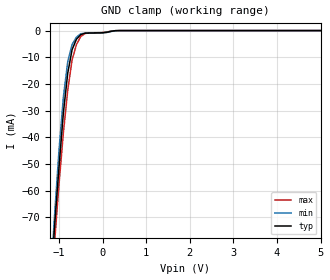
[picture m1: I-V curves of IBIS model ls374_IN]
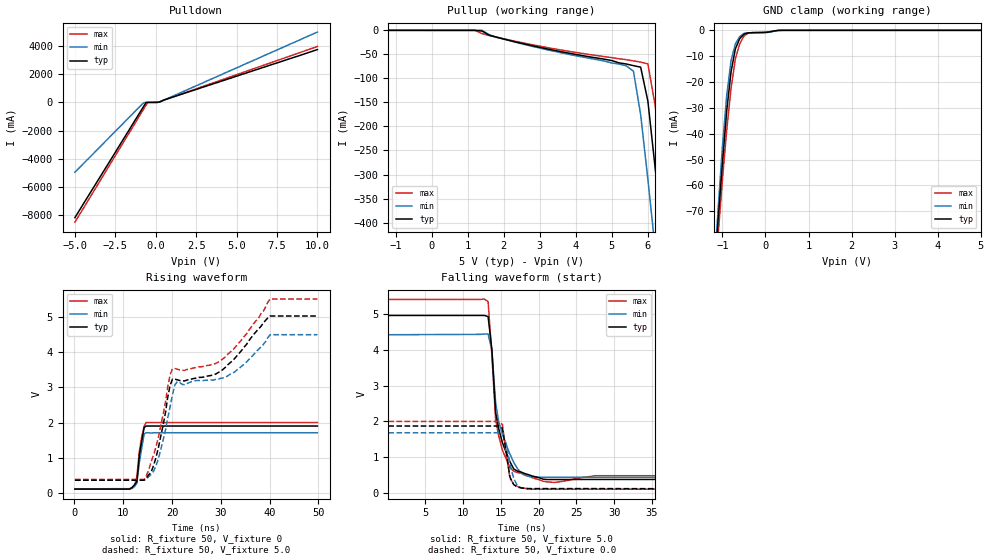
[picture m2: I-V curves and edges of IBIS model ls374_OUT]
| TEXAS INSTRUMENTS INCORPORATED
| Standard Linear and Logic Group
| IBIS Model of SN74LS374
| OCTAL D-TYPE TRANSPARENT LATCHES AND EDGE-TRIGGERED FLIP-FLOPS
| SOP 20-pin (NS), SSOP 20-pin (DB)
[IBIS Ver]   3.2
[Comment Char]  |_char
[File Name]   sn74ls374.ibs
[File Rev]   2.1 I_die
[Date]   November 18, 2004
[Source]   File originated at Texas Instruments, Inc.
[Notes]   The following is a sample IBIS file for the LS374.
   - FILE REV HISTORY
   - 2.1 Re-Release IBIS file on 11/19/04
   - Power clamp data deleted as there is no power-clamp diode
|   - All test data contained in this file are derived from
|   actual measurements.
|   - File created by Nobuhisa Ohtsubo, SLL Product Engineering.
[Disclaimer] Property of Texas Instruments Incorporated.  Unauthorized
   reproduction and/or distribution is strictly prohibited.
   This product is protected under copyright law.
   Created 2000, (C) Copyright 2000, Texas Instruments Inc.,
   All Rights Reserved.
   UNLESS THERE IS A SIGNED, WRITTEN AGREEMENT TO THE
   CONTRARY, TEXAS INSTRUMENTS () IS PROVIDING THE IBIS
   MODELS  AND WITHOUT ANY WARRANTY, EXPRESSED OR
   IMPLIED.  TI assumes no liability for:
   1) the accuracy of the IBIS models provided to your
   company;
   2) the proper functioning of these IBIS Models in your
   design or for any resulting applications; or
   3) infringement of patents, copyrights or intellectual
   property rights resulting from your use of these IBIS
   models.
   TI provides IBIS Models as a service to our customers.
   You and your company shall not distribute, sell or give
   these models to anyone else without prior written
   permission from TI.
   TI reserves the right to make changes to our products or
   to discontinue any semiconductor product or service
   without notice, and advises our customers to obtain the
   latest version of relevant information to verify, before
   placing orders, that the information being relied on is
   current.
   Please be aware that your receipt and use of the IBIS
   information provided shall serve as acceptance of these
   terms and conditions.  If you do not accept these terms,
   you should return or destroy the IBIS models and any
   other accompanying information immediately.
|   Component LS374_NS
[Component]   ls374_NS
[Manufacturer]  Texas Instruments, Inc.
[Package]
|   typ   min   max
R_pkg   0.044   0.029   0.058
L_pkg   3.666nH   2.317nH   5.115nH
C_pkg   0.548pF   0.316pF   0.725pF
[Pin]   signal_name   model_name   R_pin   L_pin   C_pin
1   OC_NOT   ls374_IN   0.058   5.115nH   0.725pF
2   1Q   ls374_OUT   0.053   4.591nH   0.724pF
3   1D   ls374_IN   0.049   3.754nH   0.572pF
4   2D   ls374_IN   0.029   2.549nH   0.388pF
5   2Q   ls374_OUT   0.031   2.317nH   0.316pF
6   3Q   ls374_OUT   0.031   2.317nH   0.316pF
7   3D   ls374_IN   0.029   2.556nH   0.399pF
8   4D   ls374_IN   0.049   3.754nH   0.579pF
9   4Q   ls374_OUT   0.053   4.591nH   0.724pF
10   GND   GND   0.058   5.115nH   0.725pF
11   CLK   ls374_IN   0.058   5.115nH   0.725pF
12   5Q   ls374_OUT   0.053   4.591nH   0.724pF
13   5D   ls374_IN   0.049   3.754nH   0.579pF
14   6D   ls374_IN   0.029   2.557nH   0.399pF
15   6Q   ls374_OUT   0.031   2.317nH   0.316pF
16   7Q   ls374_OUT   0.031   2.317nH   0.316pF
17   7D   ls374_IN   0.029   2.557nH   0.399pF
18   8D   ls374_IN   0.049   3.754nH   0.579pF
19   8Q   ls374_OUT   0.053   4.591nH   0.724pF
20   VCC   POWER   0.058   5.115nH   0.725pF
|   Component LS374_DB
[Component]   ls374_DB
[Manufacturer]  Texas Instruments, Inc.
[Package]
|   typ   min   max
R_pkg   0.040   0.035   0.051
L_pkg   3.495nH   3.035nH   4.314nH
C_pkg   0.420pF   0.346pF   0.502pF
[Pin]   signal_name   model_name   R_pin   L_pin   C_pin
1   OC_NOT   ls374_IN   0.049   4.310nH   0.502pF
2   1Q   ls374_OUT   0.048   3.903nH   0.487pF
3   1D   ls374_IN   0.035   3.189nH   0.396pF
4   2D   ls374_IN   0.035   3.036nH   0.347pF
5   2Q   ls374_OUT   0.035   3.035nH   0.367pF
6   3Q   ls374_OUT   0.035   3.035nH   0.367pF
7   3D   ls374_IN   0.035   3.036nH   0.347pF
8   4D   ls374_IN   0.035   3.189nH   0.397pF
9   4Q   ls374_OUT   0.047   3.899nH   0.488pF
10   GND   GND   0.051   4.314nH   0.500pF
11   CLK   ls374_IN   0.051   4.314nH   0.500pF
12   5Q   ls374_OUT   0.047   3.899nH   0.488pF
13   5D   ls374_IN   0.035   3.189nH   0.397pF
14   6D   ls374_IN   0.035   3.036nH   0.346pF
15   6Q   ls374_OUT   0.035   3.035nH   0.367pF
16   7Q   ls374_OUT   0.035   3.035nH   0.367pF
17   7D   ls374_IN   0.035   3.036nH   0.346pF
18   8D   ls374_IN   0.035   3.189nH   0.397pF
19   8Q   ls374_OUT   0.047   3.899nH   0.488pF
20   VCC   POWER   0.051   4.314nH   0.502pF
| Models and submodels in the file (2): ls374_IN (Input), ls374_OUT (3-state)
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|   Model LS374_IN
[Model]   ls374_IN
Model_type  Input
Polarity   Inverting
Vinl = 0.8
Vinh = 2.0
| variable   typ   min   max
C_comp   1.33pf   1.00pf   1.66pf
[Temperature Range]   25   0   70
[Voltage Range]   5.0   4.75   5.25
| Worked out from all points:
|   GND clamp passes 1 mA (typ) near -0.41 V on its own axis
[GND Clamp]
|   Voltage   I(typ)   I(min)   I(max)
-5V       -1.19A     -1.28A     -1.1A
-1.2V     -97.9mA    -94.9mA    -103mA
-1.1V     -73mA      -68.8mA    -79.1mA
-1V       -51.2mA    -44.9mA    -57.6mA
-900mV    -30.9mA    -25mA      -38.4mA
-800mV    -16mA      -11.7mA    -22.4mA
-700mV    -7.17mA    -5.25mA    -11mA
-600mV    -3.23mA    -2.46mA    -5.25mA
-500mV    -1.49mA    -1.17mA    -2.19mA
-400mV    -972uA     -958uA     -1.08mA
300mV     -31.8uA    -42.7uA    -27.7uA
5V        848pA      59.6pA     3.3nA
|   Model LS374_OUT
[Model]   ls374_OUT
Model_type  3-state
Polarity   Non-Inverting
Enable   Active-Low
Vmeas = 1.3v
Cref = 0pf
| variable   typ   min   max
C_comp   5.8pf   4.35pf   7.25pf
[Temperature Range]   25   0   70
[Voltage Range]   5.0   4.5   5.5
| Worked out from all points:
|   slope of the pulldown table from 0 to 0.75 V, typ, clamps not added: 2.87 ohm
|   GND clamp passes 1 mA (typ) near -0.41 V on its own axis
|   rising waveform, R_fixture 50, V_fixture 0: 20-80 % time 983ps typ, 1ns min, 1.02ns max; typ from 0.112 V to 1.9 V
|   falling waveform, R_fixture 50, V_fixture 5.0: 20-80 % time 1.62ns typ, 1.98ns min, 1.25ns max; typ from 4.97 V to 0.373 V
|   rising waveform, R_fixture 50, V_fixture 5.0: 20-80 % time 17.3ns typ, 17.3ns min, 18.1ns max; typ from 0.364 V to 5.02 V
|   falling waveform, R_fixture 50, V_fixture 0.0: 20-80 % time 763ps typ, 977ps min, 769ps max; typ from 1.87 V to 0.111 V
[Pulldown]
|   Voltage   I(typ)   I(min)   I(max)
-5V       -8.18A     -4.96A     -8.5A
-800mV    -386mA     -83.9mA    -577mA
-600mV    -14.5mA    -7.73mA    -200mA
-500mV    -6.86mA    -4.9mA     -11.3mA
100mV     -2.6mA     -3.4mA     -1.45mA
300mV     56.8mA     50mA       60.2mA
10V       3.74A      4.98A      3.96A
[Pullup]
|   Voltage   II(typ)   I(min)   I(max)
-5V       2.751uA    649.5nA    18.57uA
1.4V      -1.523mA   -61.48uA   -6.907mA
2.6V      -28.75mA   -29.78mA   -27.07mA
5.4V      -70.02mA   -73.84mA   -61.06mA
5.6V      -73.5mA    -85mA      -63.58mA
5.8V      -76.68mA   -175.9mA   -66.03mA
6V        -147.2mA   -309.9mA   -69.96mA
6.2V      -285.1mA   -453mA     -155.4mA
6.4V      -418.1mA   -591.7mA   -267.9mA
6.6V      -548.4mA   -727.9mA   -387.4mA
6.8V      -675.6mA   -862.2mA   -504.6mA
10V       -2.654A    -3.011A    -2.322A
[GND Clamp]
|   Voltage   I(typ)   I(min)   I(max)
-5V       -1.19A     -1.28A     -1.1A
-1.2V     -97.9mA    -94.9mA    -103mA
-1.1V     -73mA      -68.8mA    -79.1mA
-1V       -51.2mA    -44.9mA    -57.6mA
-900mV    -30.9mA    -25mA      -38.4mA
-800mV    -16mA      -11.7mA    -22.4mA
-700mV    -7.17mA    -5.25mA    -11mA
-600mV    -3.23mA    -2.46mA    -5.25mA
-500mV    -1.49mA    -1.17mA    -2.19mA
-400mV    -972uA     -958uA     -1.08mA
300mV     -31.8uA    -42.7uA    -27.7uA
5V        848pA      59.6pA     3.3nA
[Ramp]
| variable   typ   min   max
dV/dt_r   1.284/1.314n   1.056/1.149n   1.518/1.587n
dV/dt_f   2.742/1.529n   2.448/2.041n   3.042/1.254n
R_load = 50
[Rising Waveform]
R_fixture = 50
V_fixture = 0
|   Time   V(typ)   V(min)   V(max)
97.7ps    112mV      120mV      112mV
11.3ns    112mV      125mV      116mV
11.8ns    158mV      141mV      128mV
12.3ns    232mV      181mV      203mV
12.8ns    323mV      280mV      459mV
13.3ns    1.06V      862mV      1.18V
13.8ns    1.48V      1.28V      1.6V
14.3ns    1.86V      1.68V      1.9V
14.7ns    1.9V       1.71V      2V
49.8ns    1.9V       1.71V      2V
[Falling Waveform]
R_fixture = 50
V_fixture = 5.0
V_fixture_min = 4.5
V_fixture_max = 5.5
|   Time   V(typ)   V(min)   V(max)
97.7ps    4.97V      4.43V      5.42V
13.3ns    4.94V      4.45V      5.36V
13.8ns    4.02V      4V         3.87V
14.3ns    2.24V      2.52V      2.04V
14.7ns    1.8V       1.99V      1.6V
15.2ns    1.4V       1.65V      1.19V
16.7ns    665mV      848mV      603mV
17.7ns    577mV      555mV      542mV
19.6ns    446mV      436mV      389mV
49.8ns    373mV      435mV      477mV
[Rising Waveform]
R_fixture = 50
V_fixture = 5.0
V_fixture_min = 4.5
V_fixture_max = 5.5
|   Time   V(typ)   V(min)   V(max)
97.7ps    364mV      365mV      385mV
14.3ns    367mV      365mV      385mV
15.7ns    589mV      524mV      880mV
17.2ns    1.28V      970mV      1.58V
20.1ns    3.23V      2.79V      3.53V
21.1ns    3.21V      3.16V      3.51V
29.9ns    3.45V      3.25V      3.75V
34.8ns    4.14V      3.65V      4.44V
40.1ns    5.02V      4.49V      5.5V
49.8ns    5.02V      4.49V      5.5V
[Falling Waveform]
R_fixture = 50
V_fixture = 0.0
|   Time   V(typ)   V(min)   V(max)
97.7ps    1.87V      1.68V      2V
14.7ns    1.87V      1.68V      2V
15.2ns    1.81V      1.65V      1.91V
15.7ns    1.13V      1.36V      1.08V
16.2ns    432mV      791mV      404mV
16.7ns    226mV      398mV      239mV
17.2ns    155mV      187mV      177mV
17.7ns    137mV      128mV      147mV
18.7ns    111mV      120mV      100mV
49.8ns    111mV      110mV      100mV
